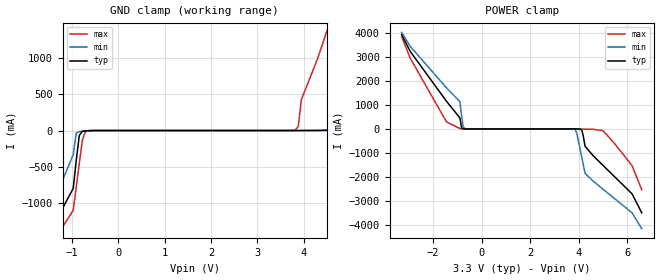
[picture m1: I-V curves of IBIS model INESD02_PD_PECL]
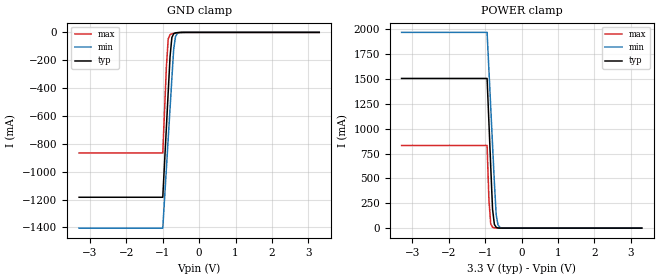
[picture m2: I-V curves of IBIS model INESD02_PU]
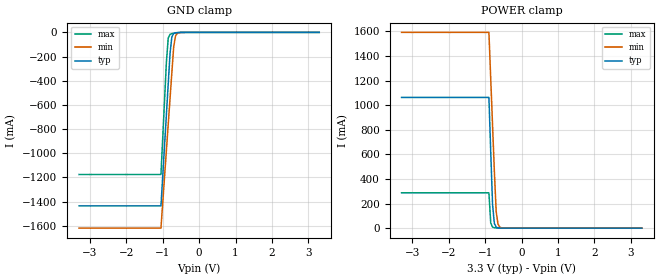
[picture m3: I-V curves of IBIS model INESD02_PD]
|   This file is an IBIS representation of the   |
|   Integrated Device Technology, Inc.   |
|   ICS874001I-05   |
|   PCI EXPRESS JITTER ATTENUATOR   |
[IBIS Ver]   4.1
[File name]   874001i_05_3v3.ibs
[File Rev]   1.0
[Date]   10 Dec 2009 | Last modified
[Source]   Originated at Integrated Device Technology, Inc.
[Disclaimer]
IDT hereby grants the user of this IBIS model a non-exclusive,
nontransferable license to use this IBIS model under the following terms.
Before using this IBIS model, the user should read this license.
If the user does not accept these terms,  the IBIS model should be
returned to IDT within 30 days.
   The user is granted this license only to use the IBIS model and
is not granted rights to sell, load, rent, lease or license the IBIS
model in whole or in part, or in modified form to anyone other than
user. User may modify the IBIS model to suit its specific
applications but rights to derivative works and such modifications
shall belong to IDT.
   This IBIS model is provided on an "AS IS" basis and IDT makes
absolutely no warranty with respect to the information contained
herein. IDT DISCLAIMS AND CUSTOMER WAIVES ALL WARRANTIES, EXPRESS
OR IMPLIED, INCLUDING WARRANTIES OF MERCHANTABILITY OR FITNESS FOR
A PARTICULAR PURPOSE. The entire risk as to quality and performance
is with the Customer. ACCORDINGLY, IN NO EVENT SHALL THE COMPANY BE
LIABLE FOR ANY DAMAGES, WHETHER IN CONTRACT OR TORT,INCLUDING ANY
LOST PROFITS OR OTHER INCIDENTAL, CONSEQUENTIAL, EXEMPLARY, OR
PUNITIVE DAMAGES ARISING OUT OF THE USE OR APPLICATION OF THE IBIS
model provided in this package. Further, IDT reserves the right to
make changes without notice to any product herein to improve
reliability, function, or design. IDT does not convey any license
under patent rights or any other intellectual property rights,
including those of third parties.
   IDT is not obligated to provide maintenance or support
for the licensed IBIS model.
[Copyright]   Copyright 2005 by Integrated Device Technology, Inc.
[Component]   ICS874001GI-05
[Manufacturer] Integrated Device Technology, Inc.
[Package]
|TSSOP 20 Lead
|   typ   min   max
R_pkg   51.85m   41.1m   62.6m
L_pkg   1.568nH   0.734nH   2.401nH
C_pkg   0.221pF   0.068pF   0.373pF
[Pin] signal_name   model_name   R_pin   L_pin   C_pin
1  PLL_SEL   INESD02_PD_PECL   62.6m   2.401n   0.373p
2  nc   nc   57.23m   1.985n   0.297p
3  nc   nc   51.85m   1.568n   0.221p
4  nc   nc   46.78m   1.151n   0.145p
5  MR   INESD02_PD_PECL   41.1m   0.734n   0.068p
6  nc   nc   41.1m   0.734n   0.068p
7  F_SEL1   INESD02_PU   46.78m   1.151n   0.145p
8  VDDA   POWER   51.85m   1.568n   0.221p
9  F_SEL0   INESD02_PD   57.23m   1.985n   0.297p
10 VDD   POWER   62.6m   2.401n   0.373p
11 OE   INESD02_PU   62.6m   2.401n   0.373p
12 CLK   INESD02_PD_PECL   57.23m   1.985n   0.297p
13 nCLK   INESD02_PU_PECL   51.85m   1.568n   0.221p
14 GND   GND   46.78m   1.151n   0.145p
15 nc   nc   41.1m   0.734n   0.068p
16 nc   nc   41.1m   0.734n   0.068p
17 nQ   ONLVDS03_LVDS01_   46.78m   1.151n   0.145p
18 Q   ONLVDS03_LVDS01_   51.85m   1.568n   0.221p
19 VDDO   POWER   57.23m   1.985n   0.297p
20 nc   nc   62.6m   2.401n   0.373p
[Diff Pin]  inv_pin  vdiff tdelay_typ tdelay_min  tdelay_max
12   13   0.15   0   0   0
18   17   NA   0   0   0
| Models and submodels in the file (5): INESD02_PD_PECL (Input), INESD02_PU (Input), INESD02_PD (Input), INESD02_PU_PECL (Input), ONLVDS03_LVDS01_ (Output)
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[Model]   INESD02_PD_PECL
Model_type  Input
Polarity   Non-Inverting
Vinl = 0.8V
Vinh = 2.0V
|   typ   min   max
C_comp   2pF   1.5pF   2.5pF
|   typ   min   max
[Voltage range]  3.3V   3.15V   3.45V
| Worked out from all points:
|   GND clamp passes 1 mA (typ) near -0.59 V on its own axis
|   POWER clamp passes 1 mA (typ) near -0.70 V on its own axis
[GND_clamp]
-3.3V     -3.894A    -4.294A    -3.674A
-1.6V     -1.569A    -1.322A    -1.74A
-974.8mV  -794.1mA   -331.5mA   -1.096A
-843.4mV  -68.33mA   -15.34mA   -452.9mA
-646.5mV  -1.912mA   -4.151mA   -2.665mA
3.818V    89.38uA    70.49uA    7.198mA
3.95V     342.2uA    75.94uA    423.8mA
4.6V      7.437mA    165.5uA    1.553A
4.9V      78.32mA    440.9uA    2.118A
5.5V      1.293A     2.769mA    3.249A
6.25V     2.651A     112.4mA    4.38A
6.6V      3.331A     896.1mA    4.946A
[POWER_clamp]
-3.3V     3.923A     4.017A     3.838A
-2.95V    3.23A      3.44A      2.951A
-1.45V    1.149A     1.709A     289.6mA
-896.9mV  456.5mA    1.133A     15.4mA
-762.9mV  4.223mA    91.07mA    1.486mA
-695.9mV  792.2uA    10.73mA    555.6uA
3.861V    -556.7uA   -26.14mA   -39.45uA
4.129V    -41.85mA   -1.19A     -4.904mA
4.263V    -724.2mA   -1.847A    -12.04mA
5V        -1.514A    -2.505A    -71.38mA
6.2V      -2.701A    -3.492A    -1.525A
6.6V      -3.492A    -4.151A    -2.536A
[Model]   INESD02_PU
Model_type   Input
Polarity   Non-Inverting
Vinl = 0.80V
Vinh = 2.0V
|   typ   min   max
C_comp   2pF   1.5pF   2.5pF
|   typ   min   max
[Voltage range]  3.3V   3.15V   3.45V
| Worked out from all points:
|   GND clamp passes 1 mA (typ) near -0.56 V on its own axis
|   POWER clamp passes 1 mA (typ) near -0.61 V on its own axis
[GND_clamp]
|Voltage   I(typ)   I(min)   I(max)
-3.3V     -1.184A    -1.405A    -865.6mA
-1V       -1.184A    -1.405A    -865.6mA
-900mV    -678.5mA   -975.1mA   -244.1mA
-850mV    -426.2mA   -760.2mA   -46.92mA
-800mV    -174mA     -545.4mA   -16.17mA
-750mV    -37.03mA   -330.8mA   -9.981mA
-700mV    -9.767mA   -120.3mA   -7.122mA
-650mV    -3.616mA   -29.78mA   -4.922mA
-600mV    -1.7mA     -7.594mA   -3.115mA
-400mV    -123.9uA   -126uA     -173.9uA
3.3V      1.866nA    3.949uA    0A
[POWER_clamp]
|Voltage   I(typ)   I(min)   I(max)
-3.3V     1.506A     1.97A      832.1mA
-950mV    1.506A     1.97A      832.1mA
-900mV    1.063A     1.592A     287.2mA
-850mV    620.4mA    1.215A     41.77mA
-800mV    191.5mA    837.4mA    8.692mA
-750mV    37.69mA    460.1mA    3.262mA
-700mV    8.032mA    133.8mA    1.662mA
-650mV    2.005mA    32.58mA    840.1uA
-600mV    607uA      8.009mA    378.6uA
-450mV    33.11uA    139.8uA    23.88uA
3.3V      -71.13uA   -77.46uA   -62.11uA
[Model]   INESD02_PD
Model_type   Input
Polarity   Non-Inverting
Vinl = 0.80V
Vinh = 2.0V
|   typ   min   max
C_comp   2pF   1.5pF   2.5pF
|   typ   min   max
[Voltage range]  3.3V   3.15V   3.45V
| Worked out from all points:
|   GND clamp passes 1 mA (typ) near -0.56 V on its own axis
|   POWER clamp passes 1 mA (typ) near -0.61 V on its own axis
[GND_clamp]
|Voltage   I(typ)   I(min)   I(max)
-3.3V     -1.436A    -1.62A     -1.176A
-1.05V    -1.436A    -1.62A     -1.176A
-900mV    -678.5mA   -975.1mA   -244mA
-850mV    -426.1mA   -760.1mA   -46.85mA
-800mV    -173.9mA   -545.4mA   -16.11mA
-750mV    -36.96mA   -330.7mA   -9.916mA
-700mV    -9.696mA   -120.2mA   -7.056mA
-650mV    -3.545mA   -29.7mA    -4.857mA
-600mV    -1.629mA   -7.52mA    -3.049mA
-400mV    -52.81uA   -52.52uA   -108.7uA
3.3V      71.13uA    77.43uA    62.11uA
[POWER_clamp]
|Voltage   I(typ)   I(min)   I(max)
-3.3V     1.063A     1.593A     287.3mA
-900mV    1.063A     1.593A     287.3mA
-850mV    620.5mA    1.215A     41.84mA
-800mV    191.6mA    837.5mA    8.757mA
-750mV    37.76mA    460.2mA    3.328mA
-700mV    8.104mA    133.8mA    1.728mA
-650mV    2.076mA    32.66mA    905.3uA
-600mV    678.1uA    8.083mA    443.8uA
-450mV    104.2uA    213.3uA    89.09uA
3.3V      -3.041nA   -3.986uA   0A
